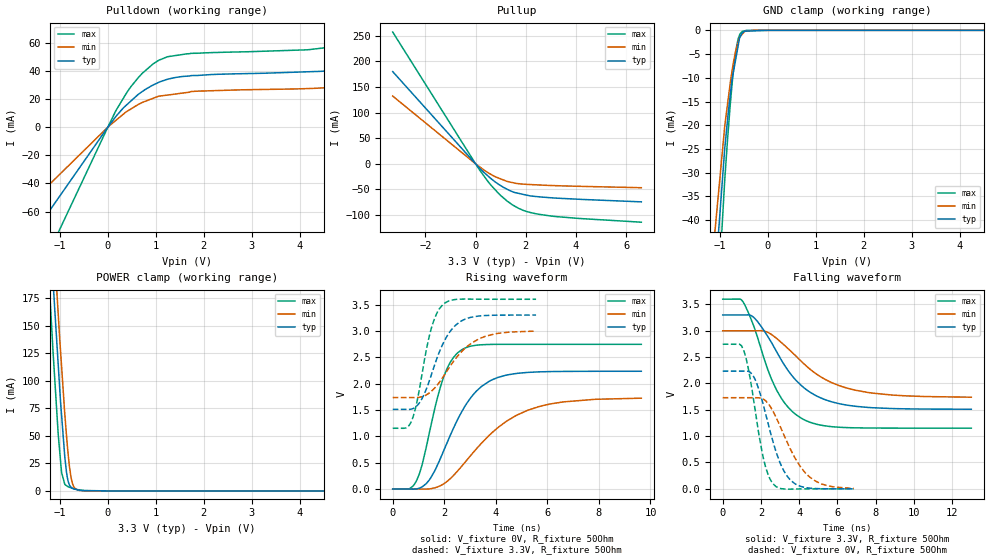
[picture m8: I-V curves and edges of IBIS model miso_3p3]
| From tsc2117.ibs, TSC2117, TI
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|   miso_3p3 Model
[Model]   miso_3p3
Model_type   3-state
Polarity   Non-Inverting
Vmeas = 1.65
Vref = 1.65
Cref = 10pF
Rref = 50
|   typ   min   max
|   (nom PVT)   (fast PVT)   (slow PVT)
|C_comp from frequency sweep method (F=25MHz)
|C_comp   4.202e-12   3.825e-12   4.497e-12
|ON state : BUFFER OUTPUT TURNED HIGH
|C_comp   4.202e-12   3.825e-12   4.497e-12
|OFF state: BUFFER IN HIGH IMPEDANCE
|C_comp   1.589e-12   1.584e-12   1.590e-12
|C_comp from LC tank measurement(L=1nH)
|Resonant Frequency(Hz)   4.030e+09   4.090e+09   3.960e+09
C_comp   1.561e-12   1.516e-12   1.617e-12
|ON state : BUFFER OUTPUT TURNED HIGH
|Resonant Frequency(Hz)   4.030e+09   4.090e+09   3.960e+09
|C_comp   1.561e-12   1.516e-12   1.617e-12
|OFF state: BUFFER IN HIGH IMPEDANCE
|Resonant Frequency(Hz)   4.400e+09   4.430e+09   4.390e+09
|C_comp   1.310e-12   1.292e-12   1.316e-12
| Where nom  PVT is Nominal Process, 3.3V, 48C
|   Fast PVT is Strong Process,  3.6V, -40C
|   Slow PVT is Weak Process,   3V, 108C
[Voltage Range]   3.3   3   3.6
|Ambient Temperature   25   85   -40
|Junction Temperature
[Temperature Range]   48   108   -40
[Pullup Reference]   3.3   3   3.6
[Pulldown Reference]   0   0   0
[Power Clamp Reference]   3.3   3   3.6
[GND Clamp Reference]   0   0   0
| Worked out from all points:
|   slope of the pulldown table from 0 to 0.495 V, typ, clamps not added: 26.1 ohm
|   slope of the pullup table from 0 to 0.495 V, typ, clamps not added: 20.8 ohm
|   GND clamp passes 1 mA (typ) near -0.56 V on its own axis
|   POWER clamp passes 1 mA (typ) near -0.64 V on its own axis
|   falling waveform, V_fixture 3.3V, R_fixture 50Ohm: 20-80 % time 2.16ns typ, 2.71ns min, 1.61ns max; typ from 3.3 V to 1.51 V
|   rising waveform, V_fixture 0V, R_fixture 50Ohm: 20-80 % time 1.39ns typ, 2.21ns min, 849ps max; typ from 0 V to 2.23 V
|   rising waveform, V_fixture 3.3V, R_fixture 50Ohm: 20-80 % time 881ps typ, 1.24ns min, 600ps max; typ from 1.51 V to 3.3 V
|   falling waveform, V_fixture 0V, R_fixture 50Ohm: 20-80 % time 1.08ns typ, 1.46ns min, 763ps max; typ from 2.23 V to 0 V
[Pulldown]
|   Voltage   I(typ)   I(min)   I(max)
-3.3V     -161.2mA   -110.2mA   -239mA
-3mV      -146.6uA   -100.2uA   -217.3uA
172.8mV   7.814mA    4.962mA    12.02mA
478.8mV   18.5mA     12.87mA    28.66mA
720mV     25.34mA    17.58mA    38.31mA
1.062V    31.82mA    21.98mA    47.5mA
1.735V    36.63mA    25.3mA     52.44mA
4.162V    39.33mA    27.4mA     54.94mA
4.507V    39.8mA     27.95mA    56.32mA
5.148V    43.41mA    30.52mA    62.67mA
5.67V     50.2mA     35.3mA     74.14mA
6.6V      76.89mA    49.14mA    117.9mA
[GND Clamp]
|   Voltage   I(typ)   I(min)   I(max)
-3.3V     -1.728A    -1.555A    -1.958A
-1.508V   -108.1mA   -86.34mA   -140.1mA
-897.6mV  -24.76mA   -20.1mA    -31.38mA
-788.4mV  -14.04mA   -11.47mA   -16.24mA
-745.8mV  -10.3mA    -8.557mA   -11.32mA
-698.4mV  -7.665mA   -5.773mA   -6.695mA
-622.8mV  -3.462mA   -2.663mA   -1.956mA
-590.7mV  -1.678mA   -1.542mA   -1.013mA
-532.8mV  -600.5uA   -812.1uA   -205.7uA
-474mV    -179.7uA   -174.4uA   -82.35uA
-285mV    -107.5uA   -1.77uA    -4.639uA
6.6V      0A         0A         0A
[Pullup]
|   Voltage   I(typ)   I(min)   I(max)
-3.3V     180mA      132.2mA    257.1mA
172.8mV   -9.066mA   -6.319mA   -12.96mA
633.6mV   -29.81mA   -21.35mA   -42.9mA
939.6mV   -40.79mA   -28.36mA   -59.08mA
1.246V    -49.52mA   -34.23mA   -72.34mA
1.554V    -56.04mA   -37.69mA   -82.56mA
1.904V    -59.8mA    -39.73mA   -91.02mA
2.473V    -64.21mA   -41.21mA   -98.18mA
4.162V    -69.36mA   -44.01mA   -106.8mA
6.6V      -74.32mA   -46.7mA    -114mA
[POWER Clamp]
|   Voltage   I(typ)   I(min)   I(max)
-3.3V     1.958A     1.976A     1.945A
-1.339V   341.9mA    389.7mA    280.9mA
-1.156V   201.8mA    248.4mA    136.7mA
-1.134V   185.3mA    231.8mA    120.6mA
-1.115V   171.1mA    218.5mA    107.6mA
-1.037V   116.3mA    162.4mA    52.94mA
-964.8mV  69.07mA    113.3mA    16.78mA
-897.6mV  31.05mA    70.07mA    6.041mA
-828mV    8.841mA    33.42mA    3.831mA
-741mV    2.422mA    7.23mA     2.378mA
-591mV    617.8uA    482.1uA    906.8uA
6.6V      0A         0A         0A
[Ramp]
R_load = 50
|   typ   min   max
dV/dt_r   1.34028/1.38902e-09   1.0375/2.22091e-09   1.64702/8.45378e-10
dV/dt_f   1.07358/2.15871e-09   0.756541/2.70356e-09   1.46874/1.61154e-09
[Falling Waveform]
V_fixture = 3.3V
V_fixture_min = 3V
V_fixture_max = 3.6V
R_fixture = 50Ohm
|   Time   V(typ)   V(min)   V(max)
0s        3.3V       3V         3.6V
1.06ns    3.3V       3V         3.552V
1.658ns   3.242V     3V         3.056V
2.334ns   2.905V     2.975V     2.288V
2.799ns   2.615V     2.861V     1.888V
3.426ns   2.242V     2.659V     1.546V
4.22ns    1.927V     2.382V     1.319V
5.549ns   1.668V     2.041V     1.186V
6.945ns   1.566V     1.872V     1.158V
13ns      1.511V     1.739V     1.152V
[Rising Waveform]
V_fixture = 0V
V_fixture_min = 0V
V_fixture_max = 0V
R_fixture = 50Ohm
|   Time   V(typ)   V(min)   V(max)
0s        2.358nV    8.101nV    828.7pV
644ps     -772.2uV   -4.804uV   4.093mV
923ps     829.6uV    -327.4uV   157.3mV
1.136ns   37.9mV     -2.294mV   450.5mV
1.411ns   165.8mV    1.337mV    1.044V
1.982ns   731.6mV    98.77mV    2.131V
2.684ns   1.472V     436.1mV    2.643V
3.743ns   2.044V     1.018V     2.742V
5.237ns   2.212V     1.494V     2.745V
9.644ns   2.234V     1.723V     2.745V
[Rising Waveform]
V_fixture = 3.3V
V_fixture_min = 3V
V_fixture_max = 3.6V
R_fixture = 50Ohm
|   Time   V(typ)   V(min)   V(max)
0s        1.51V      1.735V     1.152V
728ps     1.517V     1.735V     1.288V
932ps     1.575V     1.735V     1.634V
1.124ns   1.704V     1.749V     2.142V
1.48ns    2.138V     1.845V     3.016V
1.717ns   2.481V     1.966V     3.34V
1.99ns    2.797V     2.153V     3.518V
2.607ns   3.171V     2.572V     3.601V
3.321ns   3.281V     2.842V     3.601V
5.561ns   3.3V       2.996V     3.6V
[Falling Waveform]
V_fixture = 0V
V_fixture_min = 0V
V_fixture_max = 0V
R_fixture = 50Ohm
|   Time   V(typ)   V(min)   V(max)
0s        2.234V     1.73V      2.745V
1.091ns   2.234V     1.73V      2.635V
1.58ns    2.153V     1.73V      1.774V
2.1ns     1.625V     1.707V     625.1mV
2.379ns   1.235V     1.617V     265mV
2.676ns   838mV      1.44V      79.88mV
3.401ns   225.7mV    861mV      -6.265mV
4.358ns   22.2mV     288.6mV    -412.6uV
5.2ns     2.034mV    88.51mV    105.8uV
6.856ns   109.7uV    7.357mV    5.214uV
